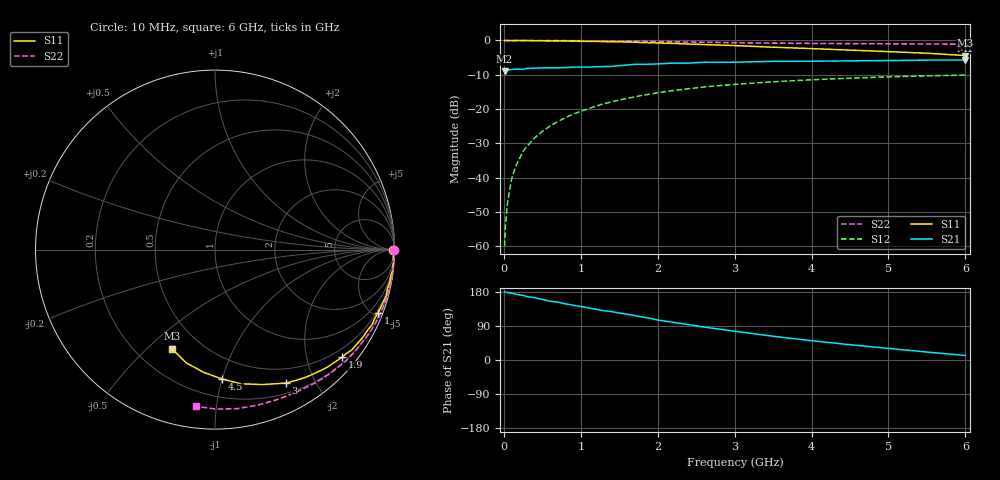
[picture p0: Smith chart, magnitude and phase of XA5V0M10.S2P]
! SIEMENS Discrete & RF Semiconductors
! BFY180
! Si NPN RF Bipolar Junction Transistor in MICRO-X
! VCE = 5 V  IC = 0.1 mA
! Common Emitter S-Parameters:  May  1997
# GHz  S  MA  R  50
!  f  S11  S21  S12  S22
! GHz  MAG  ANG  MAG  ANG  MAG  ANG  MAG  ANG
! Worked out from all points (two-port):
!   36 points, 10 MHz to 6 GHz, reference 50 ohm
!   highest |S21| = -5.71 dB at 6 GHz (marker M1); lowest = -8.9 dB at 10 MHz (marker M2)
!   |S21| within 3 dB of the highest: 16.98 MHz to end of sweep
!   lowest |S11| = -4.4 dB at 6 GHz (marker M3), VSWR 4.03, Z = 17.3 - j30 ohm
!   |S11| at or under -10 dB: nowhere
!   |S22| runs from -1.1 to 0.0 dB; largest |S21 - S12| = 0.4
!   S11 on the Smith chart (normalised r, x): 10 MHz: open; 1 GHz: 0.38, -5.32; 1.9 GHz: 0.31, -2.69; 3 GHz: 0.32, -1.62; 4.5 GHz: 0.33, -1.00; 6 GHz: 0.35, -0.60
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0.01  0.9942 -0.2  0.357 179.9  0.001 91.7  0.9983 -0.1
0.02  0.9999 -0.4  0.371 179.0  0.002 93.2  0.9999 -0.3
0.05  0.9955 -0.9  0.369 178.0  0.0045 85.4  0.9988 -0.9
0.1  0.9945 -2.0  0.378 176.4  0.0094 90.3  0.9962 -1.9
0.15  0.9941 -3.2  0.382 174.0  0.0142 88.3  0.9999 -2.8
0.25  0.994 -5.5  0.379 170.5  0.0241 85.3  0.9999 -4.7
0.4  0.9905 -8.5  0.395 164.4  0.0378 82.8  0.9986 -7.5
0.5  0.9907 -10.5  0.398 159.7  0.0472 80.6  0.9982 -9.4
0.7  0.9884 -15.1  0.399 152.6  0.0657 76.2  0.9959 -13.1
1  0.9747 -21.2  0.409 141.2  0.0927 70.3  0.9905 -18.8
1.1  0.9692 -23.1  0.409 137.5  0.1014 68.2  0.9873 -20.6
1.5  0.9551 -31.8  0.429 123.9  0.1352 60.5  0.9781 -28.0
1.7  0.9447 -36.4  0.448 117.3  0.1504 56.7  0.9694 -31.7
1.9  0.9278 -40.3  0.451 110.3  0.1647 52.8  0.9653 -35.2
2.2  0.9061 -46.3  0.467 99.5  0.1862 47.2  0.9575 -40.5
2.6  0.8725 -54.6  0.482 87.0  0.2092 40.2  0.9422 -47.0
3  0.8422 -62.0  0.482 76.0  0.2283 33.5  0.9279 -53.4
3.5  0.7972 -70.6  0.496 62.7  0.2497 26.2  0.9143 -60.6
4  0.7608 -79.2  0.498 50.9  0.267 19.0  0.9044 -67.9
4.5  0.7226 -86.7  0.504 40.4  0.2818 12.5  0.8985 -75.0
5.5  0.6509 -104.3  0.517 21.0  0.3046 -0.5  0.8881 -89.7
6  0.6023 -113.4  0.518 11.9  0.3124 -7.1  0.8801 -96.9
